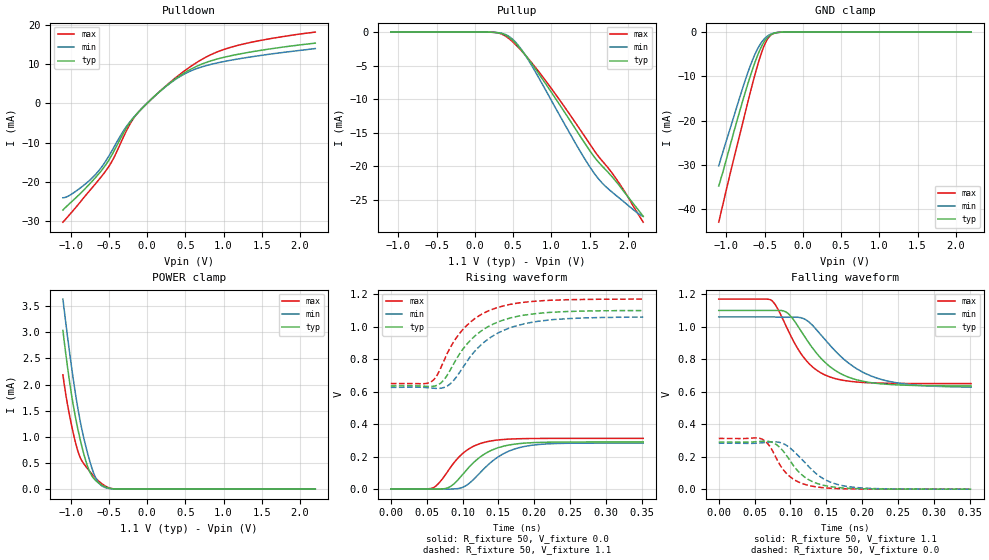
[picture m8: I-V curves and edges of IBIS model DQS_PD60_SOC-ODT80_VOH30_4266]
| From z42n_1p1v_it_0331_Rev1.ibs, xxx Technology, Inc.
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| DQS_PD60_SOC-ODT80_VOH30_4266
| (60 Ohm Pulldown, 80 Ohm System ODT Setting, VOH=VDDQ/3.0, 3200-4266Mbps)
[Model]   DQS_PD60_SOC-ODT80_VOH30_4266
Model_type   I/O
Vinl = 123.333mV
Vinh = 243.333mV
Vmeas = 183.333mV
Vref = 0.0mV
Cref = 0.0pF
Rref = 80.000Ohm
|   typ   min   max
|C_comp   0.849pF   0.799pF   0.899pF
C_comp_pullup   0.4245pF   0.3995pF   0.4495pF
C_comp_pulldown   0.4245pF   0.3995pF   0.4495pF
| Note: C_comp changes when the ODT circuit is enabled.
[Model Spec]
| Input threshold voltage corners
Vinl   0.1233V   0.1167V   0.1350V
Vinh   0.2433V   0.2367V   0.2550V
| Measurement voltage corners
Vmeas   0.1833V   0.1767V   0.1950V
| Timing spec test load voltage corners
Vref   0.0000V   0.0000V   0.0000V
| Dynamic Overshoot Parameters from LPDDR4 Specification
D_overshoot_ampl_h   0.30   NA   NA
D_overshoot_ampl_l   0.30   NA   NA
D_overshoot_area_h   0.1n   NA   NA
D_overshoot_area_l   0.1n   NA   NA
[Voltage Range]   1.1000V   1.0600V   1.1700V
[Pullup Reference]   1.1000V   1.0600V   1.1700V
| Junction Temperature (Ambient temp is 35C typ 95C min -40C max)
[Temperature Range]   50.0   110.0   -40.0
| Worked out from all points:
|   slope of the pulldown table from 0 to 0.165 V, typ, clamps not added: 55 ohm
|   slope of the pullup table from 0 to 0.165 V, typ, clamps not added: 25.9 kohm
|   GND clamp passes 1 mA (typ) near -0.45 V on its own axis
|   POWER clamp passes 1 mA (typ) near -0.88 V on its own axis
|   rising waveform, R_fixture 50, V_fixture 0.0: 20-80 % time 43.3ps typ, 46.4ps min, 37.8ps max; typ from 0 V to 0.29 V
|   falling waveform, R_fixture 50, V_fixture 1.1: 20-80 % time 53.5ps typ, 65.3ps min, 43.1ps max; typ from 1.1 V to 0.635 V
|   rising waveform, R_fixture 50, V_fixture 1.1: 20-80 % time 55.9ps typ, 59.8ps min, 52.2ps max; typ from 0.635 V to 1.1 V
|   falling waveform, R_fixture 50, V_fixture 0.0: 20-80 % time 35.2ps typ, 42.9ps min, 30.6ps max; typ from 0.29 V to 0 V
[Pulldown]
|   Voltage   I(typ)   I(min)   I(max)
-1.1V     -27.21mA   -24.07mA   -30.3mA
-905.3mV  -23.61mA   -22.06mA   -25.93mA
-654.5mV  -18.5mA    -17.72mA   -20.06mA
-469.7mV  -13.53mA   -12.46mA   -15.16mA
-275mV    -6.456mA   -6.064mA   -7.225mA
-146.3mV  -2.991mA   -2.956mA   -3.046mA
170.5mV   3.084mA    3.057mA    3.103mA
460.9mV   7.412mA    7.167mA    7.842mA
751.3mV   10.26mA    9.481mA    11.56mA
1.048V    11.92mA    10.8mA     13.99mA
1.556V    13.71mA    12.39mA    16.28mA
2.2V      15.34mA    13.95mA    18.15mA
[GND Clamp]
|   Voltage   I(typ)   I(min)   I(max)
-1.1V     -34.74mA   -30.21mA   -42.91mA
-1.05V    -31.86mA   -27.33mA   -39.27mA
-944.9mV  -25.23mA   -21.44mA   -31.55mA
-789.8mV  -15.72mA   -12.78mA   -20.72mA
-667.7mV  -8.907mA   -6.721mA   -12.29mA
-591.8mV  -5.255mA   -3.789mA   -7.493mA
-525.8mV  -2.767mA   -1.976mA   -3.963mA
-469.7mV  -1.357mA   -987.5uA   -1.789mA
-416.9mV  -597.7uA   -440.8uA   -664.7uA
-357.5mV  -192.1uA   -144.4uA   -173.8uA
-261.8mV  -18.19uA   -15.43uA   -11.09uA
2.2V      0A         0A         0A
[Pullup]
|   Voltage   I(typ)   I(min)   I(max)
-1.1V     3.138uA    4.837uA    1.415uA
233.2mV   -24.45uA   -24.33uA   -25.32uA
335.5mV   -171.1uA   -142.6uA   -234.7uA
437.8mV   -720.1uA   -591.4uA   -906.5uA
546.7mV   -1.865mA   -1.708mA   -2.036mA
678.7mV   -3.725mA   -3.812mA   -3.703mA
942.7mV   -8.017mA   -9.037mA   -7.538mA
1.312V    -14.42mA   -16.55mA   -13.5mA
1.586V    -19.01mA   -21.49mA   -18.12mA
1.698V    -20.43mA   -22.94mA   -19.69mA
1.87V     -22.66mA   -24.62mA   -22.29mA
2.2V      -27.52mA   -27.51mA   -28.38mA
[POWER Clamp]
|   Voltage   I(typ)   I(min)   I(max)
-1.1V     3.033mA    3.633mA    2.184mA
-1.041V   2.345mA    2.929mA    1.625mA
-984.5mV  1.782mA    2.31mA     1.205mA
-911.9mV  1.2mA      1.61mA     764.2uA
-852.5mV  818.5uA    1.148mA    543.6uA
-779.9mV  447.9uA    701.4uA    396.3uA
-710.6mV  232.2uA    359uA      273.1uA
-657.8mV  146.8uA    178.8uA    190.7uA
-595.1mV  80.77uA    68.34uA    109.3uA
-496.1mV  20.08uA    12.34uA    25.75uA
-393.8mV  2.22uA     1.486uA    1.931uA
2.2V      0A         0A         0A
[Ramp]
|   typ   min   max
| 20% - 80%
dV/dt_r   173.90m/43.27p   169.84m/46.36p   187.29m/37.76p
dV/dt_f   278.79m/53.47p   259.06m/65.27p   312.06m/43.11p
| 25% - 75%
|dV/dt_r   144.91m/34.53p   141.54m/37.00p   156.08m/29.98p
|dV/dt_f   232.32m/42.62p   215.88m/52.06p   260.05m/34.32p
R_load = 50
[Rising Waveform]
R_fixture = 50
V_fixture = 0.0
|   Time   V(typ)   V(min)   V(max)
0s        344.9uV    291.3uV    254.4uV
57ps      51.68uV    201.5uV    4.789mV
67ps      533.3uV    -409.3uV   36.71mV
79ps      7.179mV    -265.6uV   107.1mV
89ps      35.87mV    1.107mV    167.3mV
104ps     109.9mV    19mV       232.6mV
136ps     229.4mV    150.8mV    293.5mV
163ps     269.8mV    230.6mV    307.3mV
196ps     285.5mV    269.4mV    311.4mV
352ps     290.2mV    283.4mV    312.4mV
[Falling Waveform]
R_fixture   = 50
V_fixture   = 1.1
V_fixture_min = 1.06
V_fixture_max = 1.17
|   Time   V(typ)   V(min)   V(max)
0s        1.1V       1.06V      1.17V
74ps      1.1V       1.06V      1.161V
96ps      1.084V     1.058V     984.3mV
121ps     931mV      1.044V     797.1mV
137ps     833.7mV    979mV      731.2mV
158ps     744.4mV    871.7mV    686.2mV
192ps     673.6mV    742.3mV    659.8mV
227ps     648.1mV    675.1mV    652.5mV
276ps     638mV      640mV      650.3mV
352ps     635.3mV    628.2mV    649.9mV
[Rising Waveform]
R_fixture   = 50
V_fixture   = 1.1
V_fixture_min = 1.06
V_fixture_max = 1.17
|   Time   V(typ)   V(min)   V(max)
0s        635mV      626.1mV    649.8mV
55ps      631.5mV    622.6mV    658.1mV
64ps      638.4mV    619.8mV    697.4mV
77ps      689.9mV    630.5mV    819.7mV
89ps      782mV      676.2mV    916.2mV
105ps     886.7mV    779.3mV    1.004V
125ps     970mV      884.6mV    1.072V
148ps     1.026V     957.4mV    1.117V
220ps     1.087V     1.041V     1.162V
352ps     1.099V     1.059V     1.17V
[Falling Waveform]
R_fixture = 50
V_fixture = 0.0
|   Time   V(typ)   V(min)   V(max)
0s        290.3mV    283.5mV    312.5mV
57ps      294.1mV    284.3mV    313.4mV
75ps      287.8mV    291.4mV    236.7mV
86ps      253.6mV    286.7mV    145.3mV
97ps      191.9mV    262mV      86.31mV
113ps     100.3mV    196.9mV    40.93mV
130ps     48.07mV    118.9mV    18.71mV
154ps     17.23mV    46.78mV    6.32mV
186ps     4.672mV    13.04mV    1.688mV
352ps     425.7uV    424.8uV    278.3uV
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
